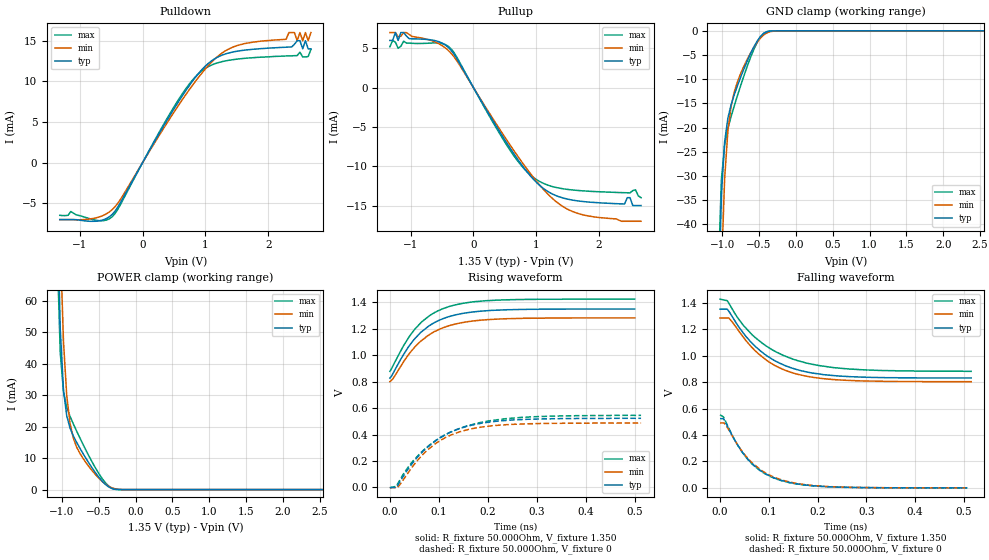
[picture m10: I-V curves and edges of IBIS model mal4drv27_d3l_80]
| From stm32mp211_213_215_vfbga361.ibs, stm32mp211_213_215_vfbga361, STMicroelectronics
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[Model] mal4drv27_d3l_80
Model_type   I/O
Polarity   Non-Inverting
Enable   Active-High
C_comp   1.684pF   1.663pF   1.711pF
C_comp_pullup   812.531fF   800.254fF   826.800fF
C_comp_pulldown   769.496fF   756.297fF   787.425fF
Vinh = 805.000mV
Vinl = 545.000mV
Vmeas = 675.000mV
Vref = 675.000mV
Rref = 50Ohms
Cref = 0pF
[Model Spec]
Vinh   805.000mV   772.000mV   855.000mV
Vinl   545.000mV   512.000mV   595.000mV
Vmeas   675.000mV   642.000mV   725.000mV
Vref   675.000mV   642.000mV   725.000mV
D_overshoot_ampl_h 0.4 NA   NA
D_overshoot_ampl_l 0.4 NA   NA
D_overshoot_area_l 110.000m NA   NA
D_overshoot_area_h 110.000m NA   NA
[Temperature Range]   25.000   125.000   -40.000
[Voltage Range]   1.350V   1.283V   1.425V
[GND Clamp Reference]   0.00V   0.00V   0.00V
[C Comp Corner]
| variable   typ   min   max
C_comp   1.684pF   1.663pF   1.711pF
C_comp_pullup   812.531fF   800.254fF   826.800fF
C_comp_pulldown   769.496fF   756.297fF   787.425fF
[Pulldown Reference]   0.00V   0.00V   0.00V
[POWER Clamp Reference]   1.350V   1.283V   1.425V
[Pullup Reference]   1.350V   1.283V   1.425V
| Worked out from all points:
|   slope of the pulldown table from 0 to 0.203 V, typ, clamps not added: 73.4 ohm
|   slope of the pullup table from 0 to 0.203 V, typ, clamps not added: 73.1 ohm
|   GND clamp passes 1 mA (typ) near -0.47 V on its own axis
|   POWER clamp passes 1 mA (typ) near -0.37 V on its own axis
|   rising waveform, R_fixture 50.000Ohm, V_fixture 1.350: 20-80 % time 73.7ps typ, 76.4ps min, 72.2ps max; typ from 0.827 V to 1.35 V
|   rising waveform, R_fixture 50.000Ohm, V_fixture 0: 20-80 % time 93.3ps typ, 85.7ps min, 106ps max; typ from -0.001 V to 0.523 V
|   falling waveform, R_fixture 50.000Ohm, V_fixture 1.350: 20-80 % time 93.8ps typ, 88.7ps min, 107ps max; typ from 1.35 V to 0.831 V
|   falling waveform, R_fixture 50.000Ohm, V_fixture 0: 20-80 % time 72.4ps typ, 75.5ps min, 71.2ps max; typ from 0.523 V to 0 V
[GND Clamp]
-1.318V   -672mA     -638mA     -661.1mA
-1.054V   -60.41mA   -84.99mA   -50.75mA
-1.011V   -34.02mA   -49.92mA   -30.84mA
-966.7mV  -22.91mA   -30.54mA   -23.58mA
-922.7mV  -18.04mA   -20.68mA   -20.16mA
-878.8mV  -15.25mA   -15.56mA   -17.69mA
-834.8mV  -13.14mA   -12.55mA   -15.44mA
-747mV    -9.486mA   -8.743mA   -11.21mA
-615.2mV  -4.709mA   -4.591mA   -5.504mA
-439.4mV  -562.2uA   -889.5uA   -546.1uA
-219.7mV  -954.1nA   -9.356uA   -215nA
2.68V     18.98nA    945nA      23.53nA
[Power Clamp]
-1.33V    889mA      842.2mA    872.8mA
-1.067V   94.44mA    130.9mA    77.96mA
-1.023V   51.04mA    78.45mA    43.53mA
-978.8mV  31.54mA    46.94mA    31.01mA
-934.8mV  23.45mA    29.85mA    26.15mA
-890.9mV  19.58mA    21.13mA    23.3mA
-847mV    17.11mA    16.47mA    20.93mA
-671.2mV  9.815mA    8.474mA    12.37mA
-495.5mV  3.823mA    3.529mA    4.955mA
-363.6mV  819.5uA    1.024mA    1.072mA
-187.9mV  4.227uA    28.6uA     2.566uA
2.668V    -29.12nA   -796.8nA   -15.73nA
[Pulldown]
-1.318V   -7mA       -7mA       -6.473mA
-483.3mV  -6.359mA   -5.772mA   -6.646mA
615.2mV   8.016mA    7.544mA    8.26mA
1.099V    12.53mA    12.37mA    12.01mA
1.626V    13.84mA    14.65mA    12.83mA
2.329V    14.22mA    16mA       13.13mA
2.461V    15mA       15mA       13.17mA
2.505V    15mA       16mA       13.58mA
2.549V    14mA       15mA       13mA
2.592V    15mA       16mA       13mA
2.636V    14mA       15mA       13.05mA
2.68V     14mA       16mA       13.93mA
[Pullup]
-1.33V    6mA        7mA        5.193mA
-1.286V   6mA        7mA        6mA
-1.199V   6mA        6.476mA    5mA
-1.111V   7mA        7mA        5.908mA
-363.6mV  4.825mA    4.437mA    4.996mA
647mV     -8.461mA   -8.049mA   -8.711mA
1.174V    -13.16mA   -13.46mA   -12.37mA
1.658V    -14.4mA    -15.99mA   -13.08mA
2.405V    -14.8mA    -17mA      -13.37mA
2.492V    -14mA      -17mA      -13.39mA
2.58V     -15mA      -17mA      -13mA
2.668V    -15mA      -17mA      -14mA
[Ramp]
R_load=50.000Ohm
dV/dt_r   312.900mV/85.000ps  290.098mV/82.000ps  327.000mV/90.500ps
dV/dt_f   312.900mV/85.000ps  290.098mV/83.000ps  327.000mV/90.500ps
[Rising waveform]
R_fixture=50.000Ohm
V_fixture=1.350
V_fixture_min=1.283
V_fixture_max=1.425
0s        827mV      801mV      878mV
7ps       866mV      826mV      925mV
31ps      1.025V     968mV      1.092V
53ps      1.135V     1.071V     1.207V
68ps      1.189V     1.122V     1.263V
83ps      1.23V      1.162V     1.305V
119ps     1.291V     1.221V     1.367V
158ps     1.322V     1.254V     1.398V
224ps     1.342V     1.275V     1.418V
500ps     1.35V      1.283V     1.425V
[Rising waveform]
R_fixture=50.000Ohm
V_fixture=0
0s        -592.9uV   -2.233mV   -3.551mV
13ps      -592.9uV   -2.233mV   8.816mV
15ps      9.671mV    -2.233mV   21.87mV
43ps      169mV      141mV      181mV
77ps      306mV      284mV      309mV
116ps     404mV      382mV      403mV
153ps     458mV      431mV      460mV
208ps     496mV      466mV      507mV
269ps     513mV      480mV      530mV
513ps     523mV      487mV      545mV
[Falling waveform]
R_fixture=50.000Ohm
V_fixture=1.350
V_fixture_min=1.283
V_fixture_max=1.425
0s        1.351V     1.284V     1.427V
15ps      1.351V     1.284V     1.415V
18ps      1.336V     1.284V     1.397V
46ps      1.179V     1.148V     1.237V
74ps      1.064V     1.03V      1.13V
111ps     964mV      928mV      1.036V
152ps     900mV      866mV      970mV
202ps     862mV      830mV      925mV
266ps     841mV      812mV      898mV
515ps     831mV      803mV      881mV
[Falling waveform]
R_fixture=50.000Ohm
V_fixture=0
0s        523mV      491mV      552mV
7ps       523mV      491mV      537mV
12ps      490mV      475mV      498mV
39ps      306mV      310mV      306mV
64ps      189mV      196mV      187mV
91ps      112mV      118mV      109mV
125ps     57.19mV    62.15mV    54.85mV
166ps     25.45mV    28.39mV    23.92mV
219ps     8.937mV    10.33mV    8.191mV
507ps     23.16uV    44.25uV    18.56uV
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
